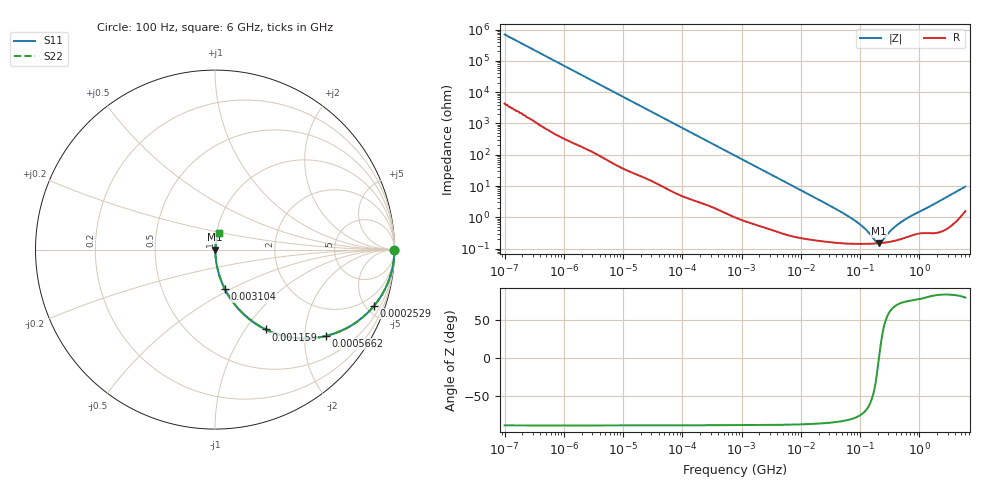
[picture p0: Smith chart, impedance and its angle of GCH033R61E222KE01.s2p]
!Murata Part Number: GCH033R61E222KE01
!These Parameters are Measured in Series Mode Connection
!Data Generated on Mar 13, 2026
!  o--ll--o
!Port1  Port2
!  o------o
!Operation Temp=25[degC], DC Bias Voltage=0[V]
!Freq. Start=100[Hz] Stop=6[GHz] 401[Steps]
# Hz S RI R 50
!Freq.(Hz) S11(Real) S11(Imag) S21(Real) S21(Imag) S12(Real) S12(Imag) S22(Real) S22(Imag)
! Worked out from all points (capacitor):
!   401 points, 100 Hz to 6 GHz, reference 50 ohm
!   read as one part in series: C = 2.27 nF near 109 Hz
!   lowest |Z| = 148 mohm at 208.8 MHz (marker M1)
!   series resonance near 208.5 MHz, so ESL is about 260 pH
!   S11 on the Smith chart (normalised r, x): 100 Hz: open; 252.9 kHz: 1.05, -5.68; 566.2 kHz: 1.03, -2.55; 1.159 MHz: 1.01, -1.25; 3.104 MHz: 1.01, -0.47; 6 GHz: 1.03, +0.19
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100  1 -0.000143  9e-07 0.000143  9e-07 0.000143  1 -0.000143
2008  1 -0.00285  2.25e-05 0.00285  2.25e-05 0.00285  1 -0.00285
40335  0.9965 -0.0564  0.00354 0.0564  0.00354 0.0564  0.9965 -0.0564
108014  0.9768 -0.1473  0.0232 0.1473  0.0232 0.1473  0.9768 -0.1473
252896  0.8875 -0.3116  0.1125 0.3116  0.1125 0.3116  0.8875 -0.3116
378399  0.7813 -0.4086  0.2187 0.4086  0.2187 0.4086  0.7813 -0.4086
566185  0.6179 -0.4809  0.3821 0.4809  0.3821 0.4809  0.6179 -0.4809
774597  0.4659 -0.4936  0.5341 0.4936  0.5341 0.4936  0.4659 -0.4936
1159002  0.2832 -0.4447  0.7168 0.4447  0.7168 0.4447  0.2832 -0.4447
1813585  0.1417 -0.3419  0.8583 0.3419  0.8583 0.3419  0.1417 -0.3419
3103719  0.0558 -0.2211  0.9442 0.2211  0.9442 0.2211  0.0558 -0.2211
6353432  0.0156 -0.1133  0.9844 0.1133  0.9844 0.1133  0.0156 -0.1133
1.555665e7  0.00409 -0.0469  0.9959 0.0469  0.9959 0.0469  0.00409 -0.0469
8.154455e7  0.00147 -0.00773  0.9985 0.00773  0.9985 0.00773  0.00147 -0.00773
1.220122e8  0.00143 -0.00401  0.9986 0.00401  0.9986 0.00401  0.00143 -0.00401
1.825626e8  0.00145 -0.000948  0.9985 0.000948  0.9985 0.000948  0.00145 -0.000948
2.088084e8  0.00148 1.17e-05  0.9985 -1.17e-05  0.9985 -1.17e-05  0.00148 1.17e-05
2.388273e8  0.00152 0.000969  0.9985 -0.000969  0.9985 -0.000969  0.00152 0.000969
3.124326e8  0.00164 0.00294  0.9984 -0.00294  0.9984 -0.00294  0.00164 0.00294
4.274388e8  0.00189 0.00545  0.9981 -0.00545  0.9981 -0.00545  0.00189 0.00545
6.395615e8  0.00245 0.00928  0.9976 -0.00928  0.9976 -0.00928  0.00245 0.00928
6e9  0.0241 0.0908  0.9759 -0.0908  0.9759 -0.0908  0.0241 0.0908
